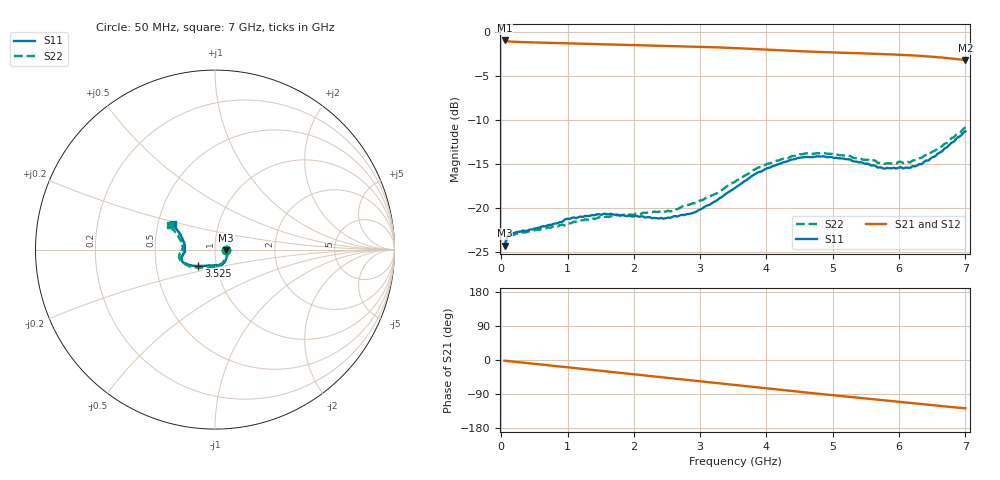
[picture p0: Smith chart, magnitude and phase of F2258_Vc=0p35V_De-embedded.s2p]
! Integrated Device Technology
! Corporate Headquarters
! 6024 Silver Creek Valley Road
! San Jose, CA 95138  USA
! Phone:  1-408-284-8200
! Toll Free:  1-800-223-1366
! Webpage:  http://www.idt.com/
! Timing and RF Division
! 515 Groton Road, Suite 102
! Westford, MA 01886-6024
! Device:  F2258
! Description: Voltage Variable RF Attenuator
! Frequency:  50.0 -  6000.00 MHz
! Package:  3x3 mm Thin QFN Plastic Package: 16 pin
! Ports:  2 RF, 2 DC
!  Pin  1  = NC
!  Pin  2  = NC
!  Pin  3  = RF2  = Port 2
!  Pin  4  = GND
!  Pin  5  = Vdd
!  Pin  6  = NC
!  Pin  7  = VCTRL
!  Pin  8  = NC
!  Pin  9  = GND
!  Pin 10  = RF1  = Port 1
!  Pin 11  = NC
!  Pin 12  = NC
!  Pin 13  = NC
!  Pin 14  = NC
!  Pin 15  = NC
!  Pin 16  = NC
! Vcntrl:  0.350 Volts
! Vdd:  +3.300 Volts
! Current:  1.089 mA
! Data:  The device was measured on a the F2258 evaluation board which has
!  individual transmission lines to the RF pins.  Data was collected
!  using a calibrated network analyzer.  The evaluation board was
!  de-embedded using a TRL calibration technique.
!  The reference plane is the edge of the package pin.
! Misc:  SN 10
!  Action Tracker AT0285
! Date Measured:  2014-12-10
! Date:  2016-01-13  MJV
! Note:
!  Integrated Device Technology supplies this data as a sample of measured
!  data at the package pin for this product.  Your particular data for this
!  product may vary.
!  Data was taken at 25 degrees C.
!  Integrated Device Technology reserves the right to change this data at anytime.
!Freq_(GHz)  S11M_(dB)  S11P_(deg)  S21M_(dB)  S21P_(deg)  S12M_(dB)  S12P_(deg)  S22M_(dB)  S22P_(deg)
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# GHz S dB R 50
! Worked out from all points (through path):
!   201 points, 50 MHz to 7 GHz, reference 50 ohm
!   highest |S21| = -1.00 dB at 50 MHz (marker M1); lowest = -3.2 dB at 7 GHz (marker M2)
!   group delay of S21, straight-line fit = 50.5 ps
!   lowest |S11| = -24.3 dB at 50 MHz (marker M3), VSWR 1.13, Z = 56.5 - j0.405 ohm
!   |S11| at or under -10 dB: start of sweep to end of sweep
!   |S22| runs from -24.3 to -10.9 dB; largest |S21 - S12| = 0.00047
!   S11 on the Smith chart (normalised r, x): 50 MHz: 1.13, -0.01; 3.525 GHz: 0.82, -0.15; 7 GHz: 0.60, +0.18
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0.05  -24.27 -3.3  -1.00 -1.9  -1.00 -1.9  -24.34 -3.1
0.08475  -23.32 -5.6  -1.07 -2.5  -1.07 -2.5  -23.41 -5.3
0.15425  -22.84 -8.8  -1.13 -3.6  -1.13 -3.6  -23.04 -9.2
0.71025  -21.93 -35.5  -1.26 -14.1  -1.26 -14.1  -22.21 -37.6
0.98825  -21.23 -49.0  -1.32 -19.3  -1.32 -19.4  -21.76 -53.4
1.2315  -21.02 -57.1  -1.37 -23.8  -1.37 -23.8  -21.40 -62.4
1.6485  -20.66 -68.7  -1.46 -31.4  -1.46 -31.4  -20.95 -75.4
2.37825  -21.20 -89.6  -1.58 -44.8  -1.58 -44.8  -20.44 -93.3
2.552  -21.12 -95.5  -1.62 -48.0  -1.62 -48.0  -20.40 -98.6
2.93425  -20.45 -112.2  -1.70 -55.1  -1.70 -55.1  -19.45 -112.0
3.525  -17.73 -135.7  -1.86 -66.2  -1.86 -66.2  -17.03 -134.9
4.0115  -15.50 -149.8  -2.04 -75.2  -2.04 -75.2  -14.99 -150.4
4.46325  -14.35 -158.4  -2.20 -83.4  -2.20 -83.4  -13.96 -161.6
4.7065  -14.22 -161.7  -2.27 -87.7  -2.28 -87.7  -13.86 -165.9
5.15825  -14.38 -167.1  -2.40 -95.6  -2.40 -95.6  -14.03 -172.8
5.64475  -15.24 -175.2  -2.51 -104.0  -2.51 -104.0  -14.65 -179.2
5.6795  -15.43 -175.2  -2.51 -104.6  -2.51 -104.6  -14.90 -179.4
5.85325  -15.50 -179.4  -2.56 -107.8  -2.57 -107.8  -14.93 175.9
6.166  -15.45 172.7  -2.67 -113.4  -2.68 -113.4  -14.84 169.9
6.33975  -15.05 166.3  -2.75 -116.5  -2.76 -116.5  -14.31 165.6
6.722  -13.13 154.3  -2.99 -123.1  -2.99 -123.1  -12.63 156.5
7  -11.30 148.7  -3.23 -127.4  -3.24 -127.4  -10.85 151.6
